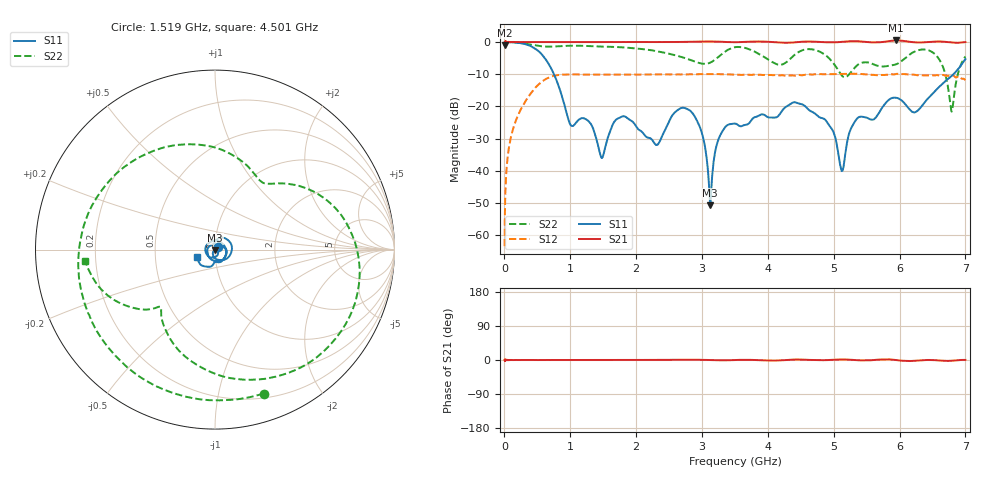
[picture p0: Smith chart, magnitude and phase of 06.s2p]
!Keysight Technologies,N5232A,MY52221221,A.10.65.11
!Date: Wednesday, October 16, 2024 11:54:02
!Correction: S11(Full 2 Port(1,4))
!S41(Full 2 Port(1,4))
!S14(Full 2 Port(1,4))
!S44(Full 2 Port(1,4))
!S2P File: Measurements: S11, S41, S14, S44:
# Hz S  RI  R 50
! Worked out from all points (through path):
!   4000 points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, 2.05 MHz to 7 GHz, reference 50 ohm
!   highest |S21| = 0.48 dB at 5.945 GHz (marker M1); lowest = -1.0 dB at 2.05 MHz (marker M2)
!   lowest |S11| = -50.7 dB at 3.126 GHz (marker M3), VSWR 1.01, Z = 50.1 - j0.283 ohm
!   |S11| at or under -10 dB: 750.9 MHz to 6.819 GHz (6.068 GHz wide, 160 % of centre)
!   |S22| runs from -21.6 to 0.0 dB; largest |S21 - S12| = 1.3
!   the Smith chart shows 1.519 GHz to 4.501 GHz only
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2049925  -0.9689 0.1506  0.8956 0.000309  0.000163 0.000659  -0.9774 0.098
1.805423e8  -0.0371 0.9771  0.997 0.000867  0.06 0.0198  -0.8138 0.5438
3.415354e8  0.8922 0.1668  0.9994 0.000541  0.0872 -0.0978  -0.4303 0.8291
4.867792e8  0.2808 -0.7088  0.9992 -0.00124  -0.0805 -0.1876  -0.0502 0.8786
6.320229e8  -0.4585 -0.2595  0.9969 0.000298  -0.2678 0.0101  0.2695 0.8045
1.16925e9  0.0308 0.0581  0.9973 0.00335  0.1632 -0.2656  0.8444 -0.2199
1.478987e9  0.0159 0.00134  0.9982 0.00311  -0.3115 0.0117  0.3589 -0.7692
1.690728e9  0.0616 -0.00304  0.9985 0.00352  -0.0255 0.3101  -0.1341 -0.8255
2.3347e9  0.000143 0.026  0.998 0.00511  -0.2852 -0.1301  -0.6385 0.3208
2.824679e9  0.072 -0.0451  1.008 0.0125  0.3042 0.0832  0.1226 0.5113
3.125666e9  0.000713 -0.00283  1.019 -0.00244  -0.0611 -0.3118  0.3071 0.3665
3.5019e9  -0.0533 0.00949  0.9929 -0.00159  -0.1221 0.285  0.7928 -0.2472
3.795887e9  0.0647 -0.0202  1.016 0.000778  0.3113 0.00342  0.0565 -0.71
4.261367e9  -0.0218 -0.0938  0.9737 -0.00551  -0.3 -0.0118  -0.3384 -0.3273
4.66735e9  -0.0813 0.0167  1.015 -0.00259  0.2764 0.1449  -0.6124 0.4653
5.12583e9  0.00882 -0.00471  1.005 0.025  -0.2779 -0.1578  0.1565 0.2559
5.437317e9  -0.0636 0.0269  1.015 -0.0205  0.0188 0.3179  0.3788 0.2923
5.83455e9  -0.0847 0.0932  1.029 0.0311  0.127 -0.2839  0.3993 -0.1541
5.944795e9  -0.045 0.1288  1.056 -0.000773  -0.1071 -0.3007  0.3787 -0.2409
6.494272e9  0.00804 0.1549  1.011 -0.00348  0.2658 0.1492  -0.6377 -0.2879
6.791759e9  0.2874 -0.0757  0.9816 -0.0329  -0.0277 -0.2996  -0.0832 -0.0036
7e9  -0.4444 -0.31  0.997 0.00452  -0.2502 0.0528  -0.5954 -0.035
